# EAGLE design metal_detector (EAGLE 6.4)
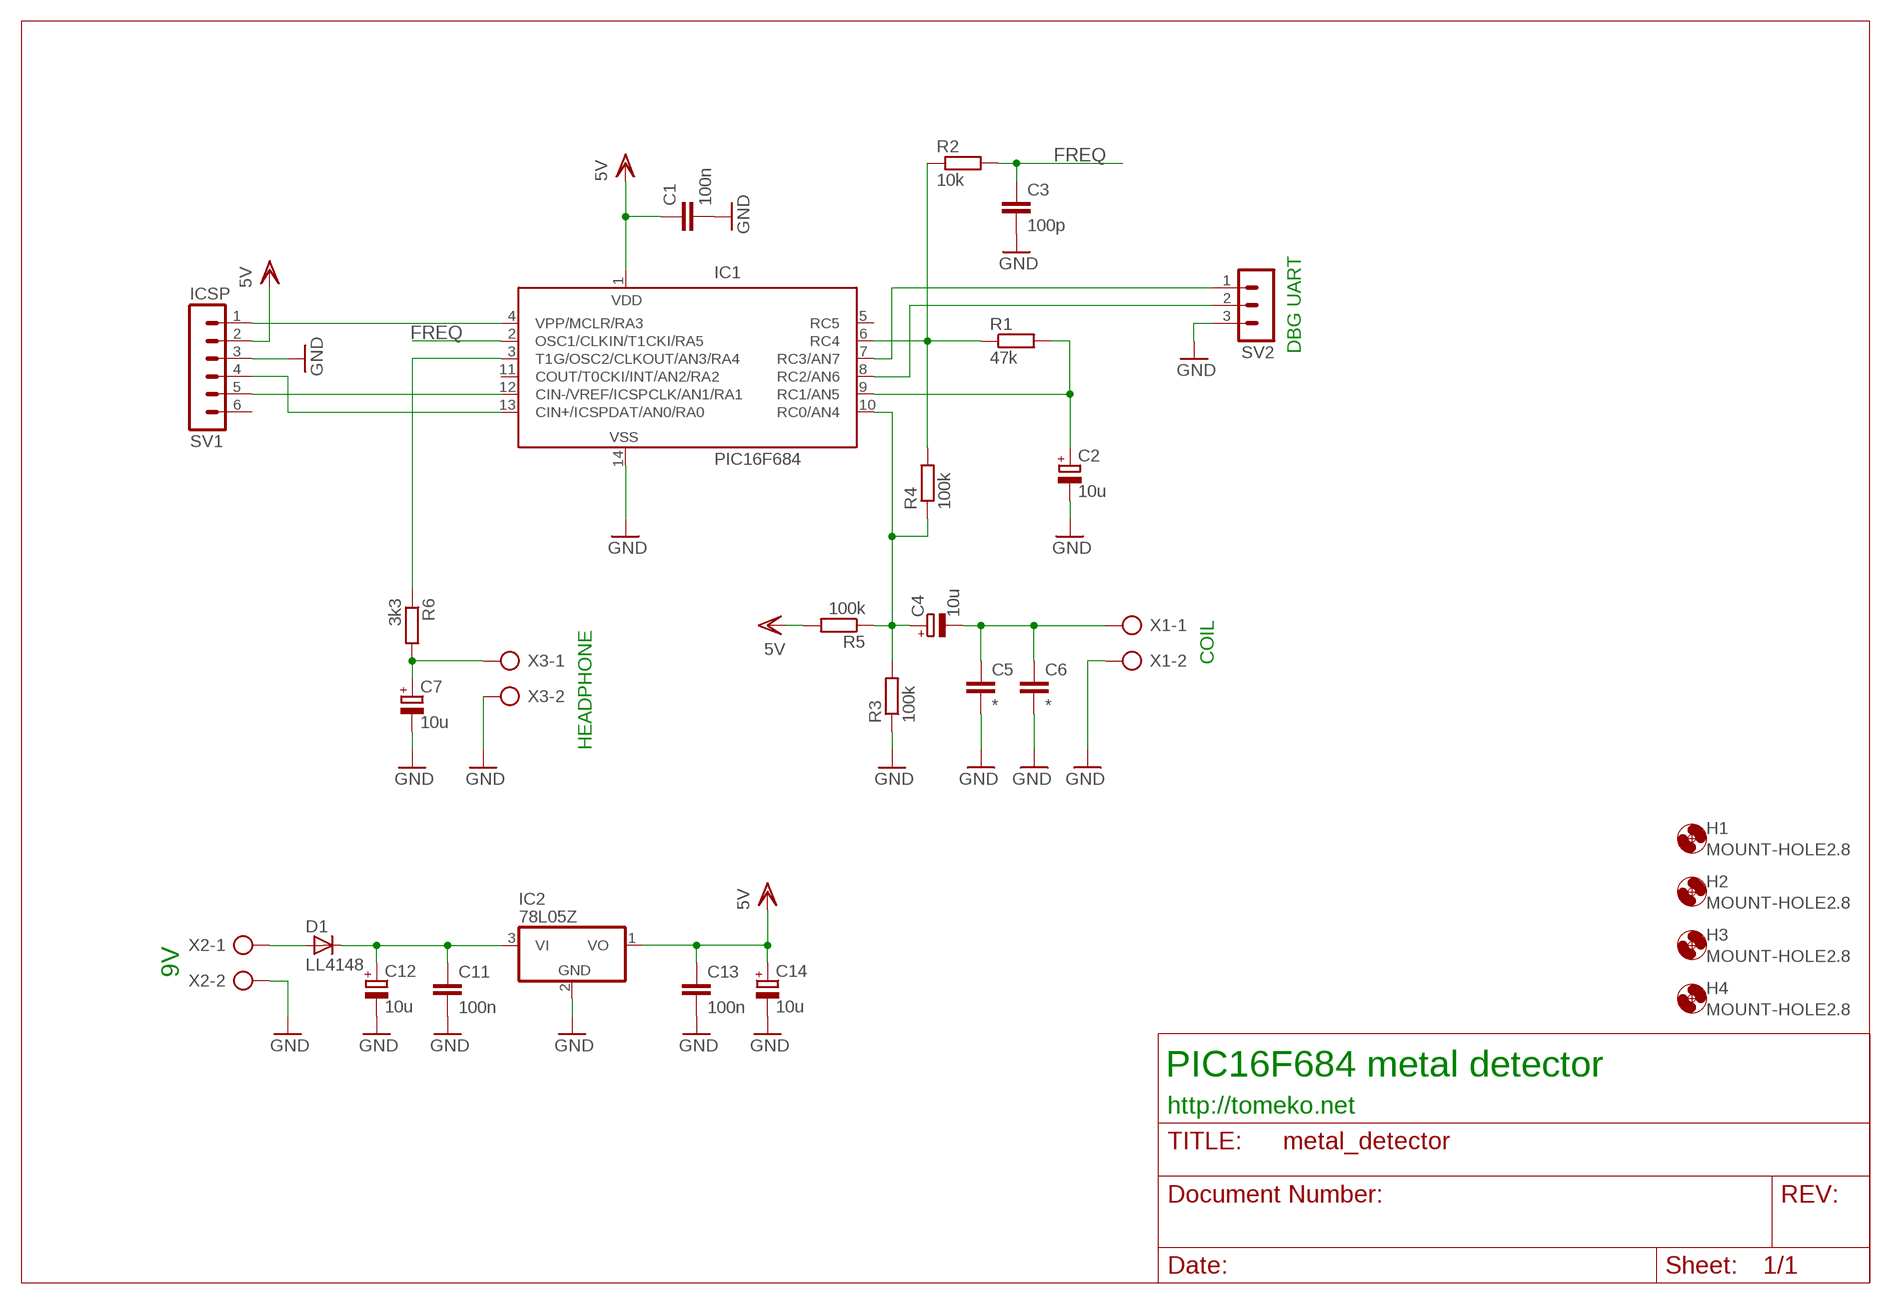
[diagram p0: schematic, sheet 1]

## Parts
C1  100n  C-0805  [C0805]
C2  10u  CPOL-EUE2.5-6  [E2,5-6]
C3  100p  C-0805  [C0805]
C4  10u  CPOL-EUE2.5-6  [E2,5-6]
C5  *  C5/3.5  [C5B3.5]
C6  *  C5/3.5  [C5B3.5]
C7  10u  CPOL-EUE2.5-6  [E2,5-6]
C11  100n  C-0805  [C0805]
C12  10u  CPOL-EUE2.5-6  [E2,5-6]
C13  100n  C-0805  [C0805]
C14  10u  CPOL-EUE2.5-6  [E2,5-6]
D1  LL4148  D-SOD-80  [SOD80]
H1  MOUNT-HOLE2.8  [2,8]
H2  MOUNT-HOLE2.8  [2,8]
H3  MOUNT-HOLE2.8  [2,8]
H4  MOUNT-HOLE2.8  [2,8]
IC1  PIC16F684  PIC16F676P  [DIL14]
IC2  78L05Z  [TO92]
R1  47k  R-EU_R0805  [R0805]
R2  10k  R-EU_R0805  [R0805]
R3  100k  R-EU_R0805  [R0805]
R4  100k  R-EU_R0805  [R0805]
R5  100k  R-EU_R0805  [R0805]
R6  3k3  R-EU_R0805  [R0805]
SV1  ICSP  MA06-1  [MA06-1]
SV2  MA03-1  [MA03-1]
X1  AK500/2  [AK500/2]
X2  AK500/2  [AK500/2]
X3  AK500/2  [AK500/2]

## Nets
FREQ: C3.1 IC1.2(OSC1/CLKIN/T1CKI/RA5) R2.2
GND: C1.2 C2.- C3.2 C5.2 C6.2 C7.- C11.2 C12.- C13.2 C14.- IC1.14(VSS) IC2.2(GND) R3.1 SV1.3 SV2.3 X1.2 X2.2 X3.2
N$1: D1.2(A) X2.1
N$2: C2.+ IC1.9(RC1/AN5) R1.2
N$3: IC1.4(VPP/MCLR/RA3) SV1.1
N$4: IC1.6(RC4) R1.1 R2.1 R4.2
N$5: C4.+ IC1.10(RC0/AN4) R3.2 R4.1 R5.1
N$6: IC1.12(CIN-/VREF/ICSPCLK/AN1/RA1) SV1.5
N$7: IC1.13(CIN+/ICSPDAT/AN0/RA0) SV1.4
N$8: IC1.7(RC3/AN7) SV2.1
N$9: IC1.3(T1G/OSC2/CLKOUT/AN3/RA4) R6.1
N$10: C4.- C5.1 C6.1 X1.1
N$11: C7.+ R6.2 X3.1
N$12: IC1.8(RC2/AN6) SV2.2
N$16: C11.1 C12.+ D1.1(C) IC2.3(VI)
VDD: C1.1 C13.1 C14.+ IC1.1(VDD) IC2.1(VO) R5.2 SV1.2 ; supply symbol labelled 5V
Unconnected: IC1.5(RC5) IC1.11(COUT/T0CKI/INT/AN2/RA2) SV1.6

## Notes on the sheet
- DBG UART
- COIL
- HEADPHONE
- 9V
- PIC16F684 metal detector
- http://tomeko.net

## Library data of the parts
C1 C3 C11 C13 = quantum-sensor:C: Capacitor
C2 C4 C7 C12 C14 = rcl:CPOL-EU: POLARIZED CAPACITOR, European symbol
C5 C6 = capacitor-wima:C: CAPACITOR
D1 = semicon-smd-ipc:D-: DIODE
H1-H4 = holes:MOUNT-HOLE: MOUNTING HOLE with drill center marker
IC1 = microchip:PIC16F676: 14-Pin, Flash-Based 8-Bit CMOS Microcontroller High Performance RISC CPU: * Only 35 instructions to learn - All single-cycle instructions except branches * Operating speed: - DC - 20 MHz oscillator/clock input - DC - 200 ns instruction cycle * Internal and external oscillator options - Precision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; MF: MICROCHIP; MPN: PIC16F676-I/P; OC_FARNELL: 9760512; OC_NEWARK: 54K2829
IC2 = linear:78*: Positive VOLTAGE REGULATOR Source: http://cache.national.com/ds/LM/LM78L05.pdf http://www.fairchildsemi.com/ds/LM/LM7805.pdf
R1-R6 = rcl:R-EU_: RESISTOR, European symbol
SV1 = con-lstb:MA06-1: PIN HEADER
SV2 = con-lstb:MA03-1: PIN HEADER; OC_FARNELL: unknown; OC_NEWARK: unknown
X1-X3 = con-ptr500:AK500/2: CONNECTOR

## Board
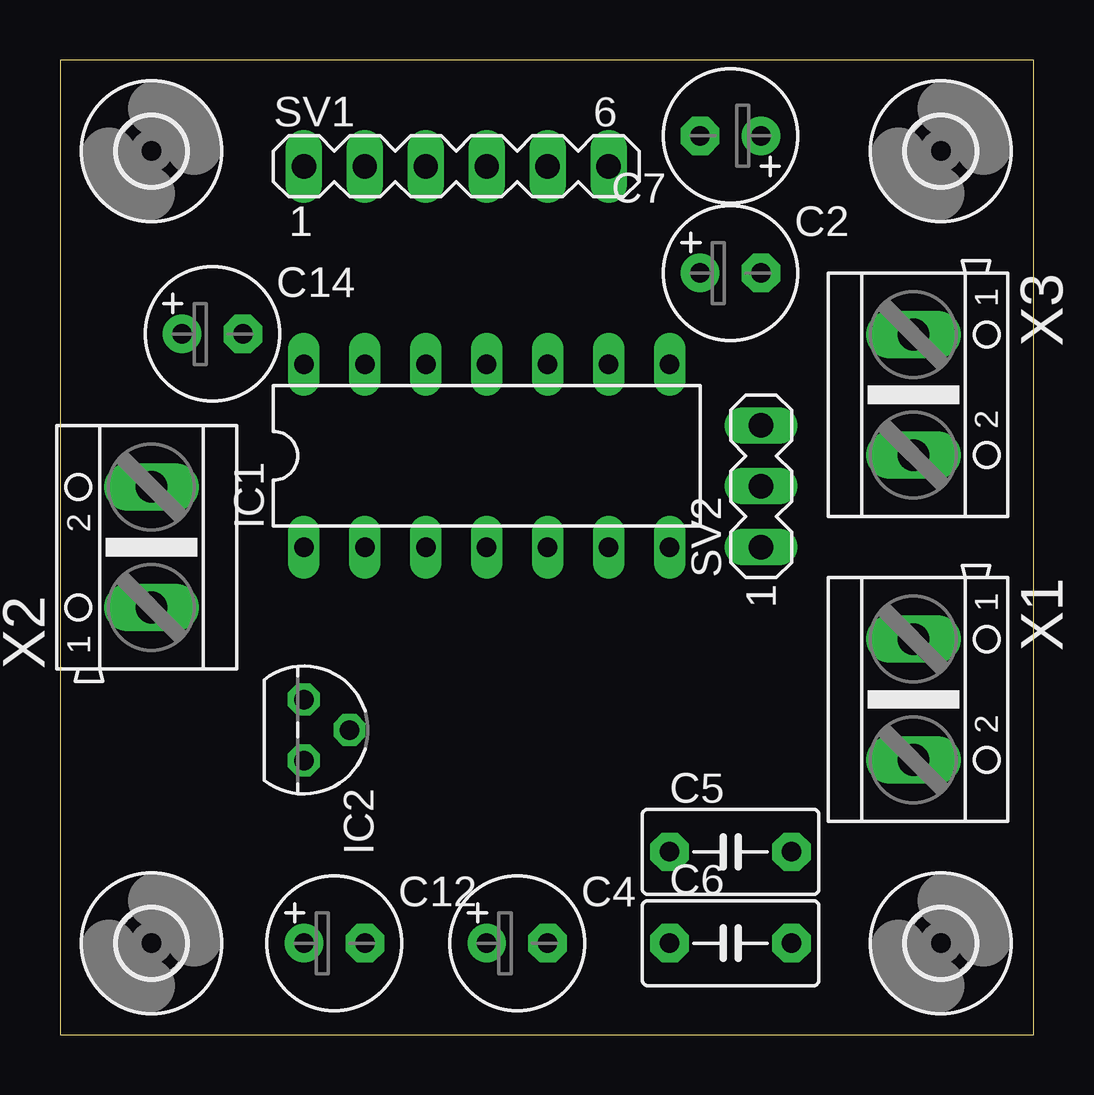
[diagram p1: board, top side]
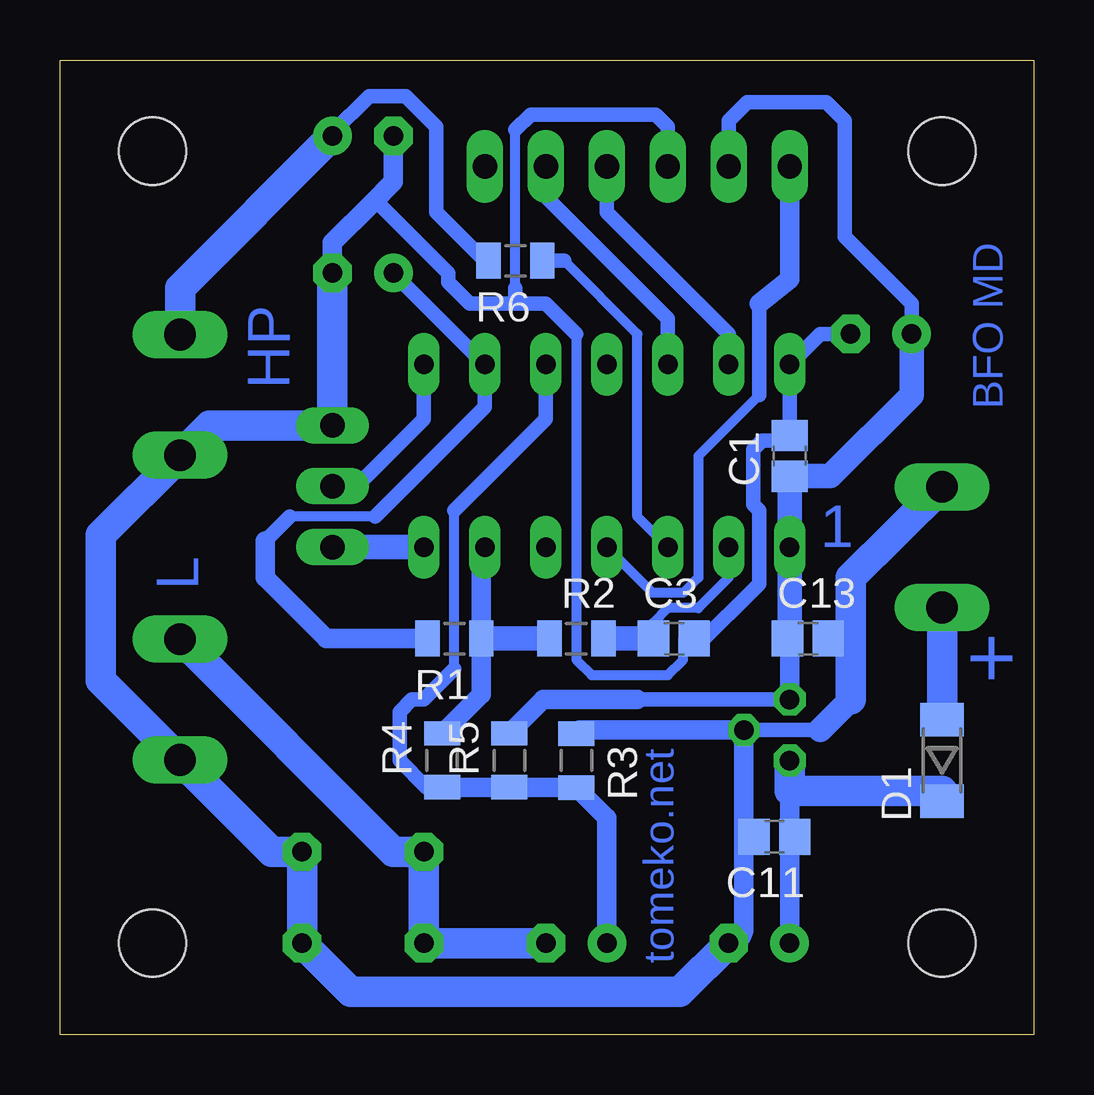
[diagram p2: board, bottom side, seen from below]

Size 40.56 x 40.63 mm. Coordinates in mm from the lower left corner, seen from the top.
Outline: 0,0 40.56,0 40.56,40.63 0,40.63 0,0
Copper layers (1*16): Top 0.035mm / dielectric 1.5mm / Bottom 0.035mm
Design rules "default": minimum track width 10mil, minimum drill 24mil, track to track 8mil, track to pad 8mil, pad to pad 8mil, via to via 8mil, smd to smd 8mil, copper to edge 40mil, drill to drill 8mil, minimum pad ring 10mil, minimum via ring 8mil, stop-mask expansion 4mil, vias tented up to drill 0mil, thermal gap 10mil

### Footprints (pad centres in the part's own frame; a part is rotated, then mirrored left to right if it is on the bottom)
C0805 = smd 1.3 x 1.5: 1 -0.85,0; 2 0.85,0
E2,5-6 = drill 0.813 pad 1.6: + -1.27,0 | drill 0.813 pad 1.6 octagon: - 1.27,0
C5B3.5 = drill 0.813 pad 1.6 octagon: 1 -2.54,0; 2 2.54,0
SOD80 = smd 1.4 x 1.8: 1 -1.7,0; 2 1.7,0
2,8 = hole 2.8: 0,0
DIL14 = drill 0.813 long: 1 -7.62,-3.81; 2 -5.08,-3.81; 3 -2.54,-3.81; 4 0,-3.81; 5 2.54,-3.81; 6 5.08,-3.81; 7 7.62,-3.81; 8 7.62,3.81; 9 5.08,3.81; 10 2.54,3.81; 11 0,3.81; 12 -2.54,3.81; 13 -5.08,3.81; 14 -7.62,3.81
TO92 = drill 0.813 octagon: 1 -1.27,0; 2 0,1.905; 3 1.27,0
R0805 = smd 1.016 x 1.5: 1 -1.118,0; 2 1.128,0
MA06-1 = drill 1.016 long: 1 -6.35,0; 2 -3.81,0; 3 -1.27,0; 4 1.27,0; 5 3.81,0; 6 6.35,0
MA03-1 = drill 1.016 long: 1 -2.54,0; 2 0,0; 3 2.54,0
AK500/2 = drill 1.321 long: 1 -2.515,0; 2 2.515,0

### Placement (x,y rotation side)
C1  10.16,24.13 90 bottom
C2  27.94,31.75 0 top
C3  14.99,16.51 0 bottom
C4  19.05,3.81 0 top
C5  27.94,7.62 0 top
C6  27.94,3.81 0 top
C7  27.94,37.47 180 top
C11  10.79,8.26 180 bottom
C12  11.43,3.81 0 top
C13  9.4,16.51 0 bottom
C14  6.35,29.21 0 top
D1  3.81,11.43 90 bottom
H1  3.81,36.83 0 top
H2  36.7,3.81 0 top
H3  3.81,3.81 0 top
H4  36.7,36.83 0 top
IC1  17.78,24.13 0 top
IC2  10.16,12.7 270 top
R1  24.13,16.51 180 bottom
R2  19.05,16.51 0 bottom
R3  19.05,11.43 270 bottom
R4  24.64,11.43 90 bottom
R5  21.84,11.43 90 bottom
R6  21.59,32.26 180 bottom
SV1  16.51,36.2 0 top
SV2  29.21,22.86 90 top
X1  35.56,13.97 270 top
X2  3.81,20.32 90 top
X3  35.56,26.67 270 top

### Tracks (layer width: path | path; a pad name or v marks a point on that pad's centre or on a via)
FREQ
  Bottom 0.254: 15.88,16.51 C3.1
  Bottom 0.406: 15.88,16.51 15.88,17.14 15.24,17.78 13.97,17.78 12.7,19.05 IC1.2
  Bottom 1.016: R2.2 C3.1
GND
  Bottom 0.254: 14.61,16.51 C3.2 | 35.56,11.43 X1.2
  Bottom 0.406: 21.59,31.11 21.59,37.72 | 14.61,16.51 14.61,15.62 15.24,14.99 18.41,14.99 19.05,15.62 19.05,29.21
  Bottom 0.46: C13.2 7.62,16.51
  Bottom 0.61: C1.2 IC1.14 8.89,29.21 C14.- | 21.59,37.72 20.95,38.35 15.75,38.35 15.24,37.85 SV1.3 | 19.05,29.21 20.32,30.48 21.59,30.48 | 21.59,30.48 23.5,30.48 24.38,31.37 24.38,31.75 27.3,34.67 27.56,34.67 | 8.89,12.7 IC2.2 | 10.16,24.77 11.3,24.77 11.68,24.38 11.68,22.1 11.43,21.84 11.43,18.8 11.77,18.45 13.72,16.51 C3.2 | 21.59,31.11 21.59,30.48
  Bottom 0.813: C11.2 12.06,8.68 IC2.2 | IC2.2 12.06,4.45 arc90 C12.- | 10.16,24.77 C1.2 | C7.- 26.67,35.56 27.56,34.67 29.21,33.02 C2.- | IC2.2 18.9,12.7 R3.1
  Bottom 1.016: 7.62,13.97 8.89,12.7
  Bottom 1.27: X2.2 7.62,19.05 7.62,16.51 7.62,13.97 | C12.- 14.73,1.78 28.45,1.78 C6.2 C5.2 31.75,7.62 35.56,11.43 | X1.2 38.86,14.76 38.86,20.83 35.56,24.13 X3.2 34.31,25.4 SV2.3 C2.-
N$1
  Bottom 1.27: X2.1 D1.2
N$2
  Bottom 0.406: 27.43,21.59 30.99,21.59
  Bottom 0.61: C2.+ IC1.9 22.86,26.16 27.43,21.59 | 30.99,21.59 32,20.57
  Bottom 0.813: 32,20.57 32,19.05 29.46,16.51 R1.2
N$3
  Bottom 0.406: IC1.4 15.88,18.41 14.61,18.41 13.97,19.05 13.97,24.13 11.43,26.67
  Bottom 0.61: 11.43,26.67 11.43,30.48
  Bottom 0.813: SV1.1 10.16,31.5 11.43,30.48
N$4
  Bottom 0.254: 22.86,16.51 R1.1
  Bottom 0.813: IC1.6 23.01,20.17 R1.1 23.01,14.18 R4.2
  Bottom 1.016: R2.1 R1.1
N$5
  Bottom 0.406: 24.13,15.24 24.13,21.84
  Bottom 0.61: IC1.10 20.32,25.65 24.13,21.84 | 24.13,15.24 25.4,13.97 25.91,13.97 26.42,13.46 26.42,11.43 25.3,10.31 R4.1
  Bottom 0.813: C4.+ 17.78,9.03 R3.2 19.06,10.31 R5.1 R4.1
N$6
  Bottom 0.61: IC1.12 15.24,29.84 20.32,34.92 SV1.5
N$7
  Bottom 0.61: IC1.13 12.7,29.21 17.78,34.29 SV1.4
N$8
  Bottom 1.016: SV2.1 IC1.7
N$9
  Bottom 0.406: 19.56,32.26 16.51,29.21 16.51,21.59 IC1.3
  Bottom 0.61: 19.56,32.26 R6.1
N$10
  Bottom 1.27: C4.- C6.1 C5.1 26.67,7.62 35.53,16.48 X1.1
N$11
  Bottom 0.254: 22.86,32.26 R6.2
  Bottom 0.61: 22.86,32.26 24.89,34.29 24.89,37.85 26.16,39.12 27.69,39.12 29.21,37.59 C7.+
  Bottom 1.27: C7.+ 35.56,31.11 X3.1
N$12
  Bottom 0.61: IC1.8 25.4,25.65 28.19,22.86 SV2.2
N$16
  Bottom 0.254: 3.81,10.16 D1.1 | 10.16,8.26 C11.1
  Bottom 0.813: 10.16,10.16 10.16,8.26 C12.+
  Bottom 1.27: IC2.3 10.16,10.16 3.81,10.16
VDD
  Bottom 0.254: 10.16,22.86 C1.1 | 10.16,16.51 C13.1
  Bottom 0.61: 16.51,13.97 IC2.1 | C14.+ 5.08,30.48 7.87,33.27 7.87,38.1 8.64,38.86 11.94,38.86 12.7,38.1 SV1.2
  Bottom 0.813: R5.2 20.43,13.97 16.51,13.97 | 10.07,14.06 IC2.1 10.16,16.42 C13.1
  Bottom 1.016: 10.16,22.86 IC1.1 10.16,16.51 | C14.+ 5.08,26.67 8.47,23.28 C1.1

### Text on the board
Bottom: BFO MD | HP | 1 | L | + | tomeko.net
